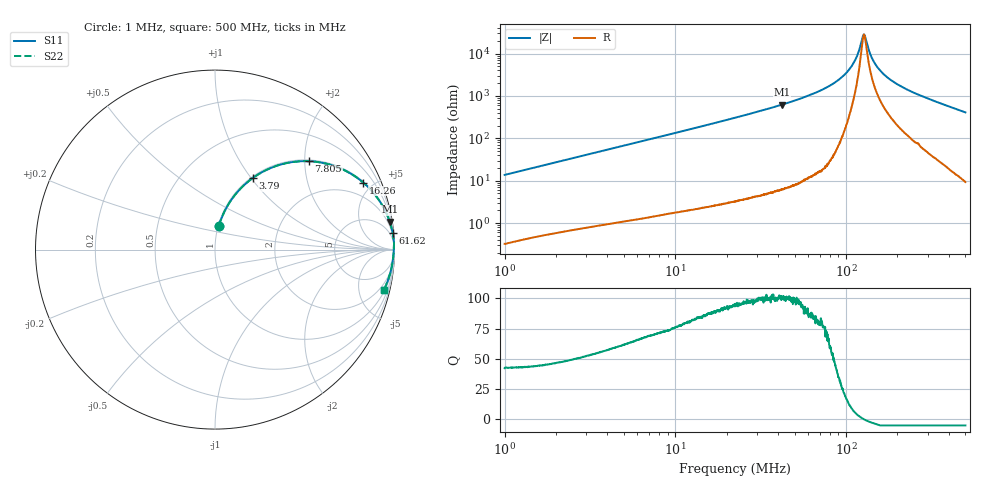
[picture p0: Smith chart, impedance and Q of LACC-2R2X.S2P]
!s-Parameter Generated by FASTRON Sdn. Bhd.
!FASTRON P/N : LACC-2R2X
!Keysight Technologies,E4991B,MY54100416,A.01.15
!Date: Wed Mar 18 09:04:33 2026
!Version  : Rev00 Wed Mar 18 09:04:33 2026
!Data & Calibration Information:
!PortZ  Port1:50+j0  Port2:50+j0
!When reading, reference impedance value at option line is always used.
!Remarks : This data is being provided solely for informational purposes.
!Freq	S11	S21	S12	S22
# Hz S dB R 50
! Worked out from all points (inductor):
!   1601 points, 1 MHz to 500 MHz, reference 50 ohm
!   read as one part in series: L = 2.17 uH near 1.032 MHz
!   highest Q = 101 at 42.12 MHz (marker M1), where L = 2.36 uH
!   self-resonance near 127.4 MHz
!   S11 on the Smith chart (normalised r, x): 1 MHz: 1.01, +0.27; 3.79 MHz: 1.02, +1.02; 7.805 MHz: 1.03, +2.09; 16.26 MHz: 1.05, +4.40; 61.62 MHz: 1, +21; 500 MHz: 1.19, -8.20
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1000000  -17.36 80.9  -0.11 -7.8  -0.11 -7.8  -17.36 80.9
2820919  -9.02 68.2  -0.64 -20.7  -0.64 -20.7  -9.02 68.2
3789585  -6.91 62.2  -1.07 -26.8  -1.07 -26.8  -6.91 62.2
7804534  -2.88 43.3  -3.27 -45.9  -3.27 -45.9  -2.88 43.3
7957584  -2.80 42.8  -3.36 -46.4  -3.36 -46.4  -2.80 42.8
1.626158e7  -0.85 24.4  -7.69 -65.0  -7.69 -65.0  -0.85 24.4
2.236068e7  -0.47 18.0  -10.18 -71.3  -10.18 -71.3  -0.47 18.0
4.211556e7  -0.12 9.1  -16.02 -80.3  -16.02 -80.3  -0.12 9.1
6.162465e7  -0.05 5.4  -20.53 -83.9  -20.53 -83.9  -0.05 5.4
6.307767e7  -0.04 5.2  -20.85 -84.1  -20.85 -84.1  -0.04 5.2
8.310792e7  -0.02 3.0  -25.60 -85.9  -25.60 -85.9  -0.02 3.0
1.009219e8  -0.02 1.6  -31.13 -85.0  -31.13 -85.0  -0.02 1.6
1.133942e8  -0.02 0.8  -37.15 -78.5  -37.15 -78.5  -0.02 0.8
1.239906e8  -0.03 0.2  -46.61 -44.4  -46.61 -44.4  -0.03 0.2
1.269141e8  -0.03 0.0  -49.06 -9.0  -49.06 -9.0  -0.03 0.0
1.299065e8  -0.03 -0.1  -47.49 28.6  -47.49 28.6  -0.03 -0.1
1.387738e8  -0.04 -0.5  -39.63 65.8  -39.63 65.8  -0.04 -0.5
1.470992e8  -0.04 -0.9  -35.53 73.3  -35.53 73.3  -0.04 -0.9
1.602216e8  -0.05 -1.5  -31.56 77.6  -31.56 77.6  -0.05 -1.5
1.77937e8  -0.05 -2.2  -28.30 79.7  -28.30 79.7  -0.05 -2.2
2.553547e8  -0.09 -5.0  -21.25 81.0  -21.25 81.0  -0.09 -5.0
5e8  -0.30 -13.6  -12.55 75.1  -12.55 75.1  -0.30 -13.6
